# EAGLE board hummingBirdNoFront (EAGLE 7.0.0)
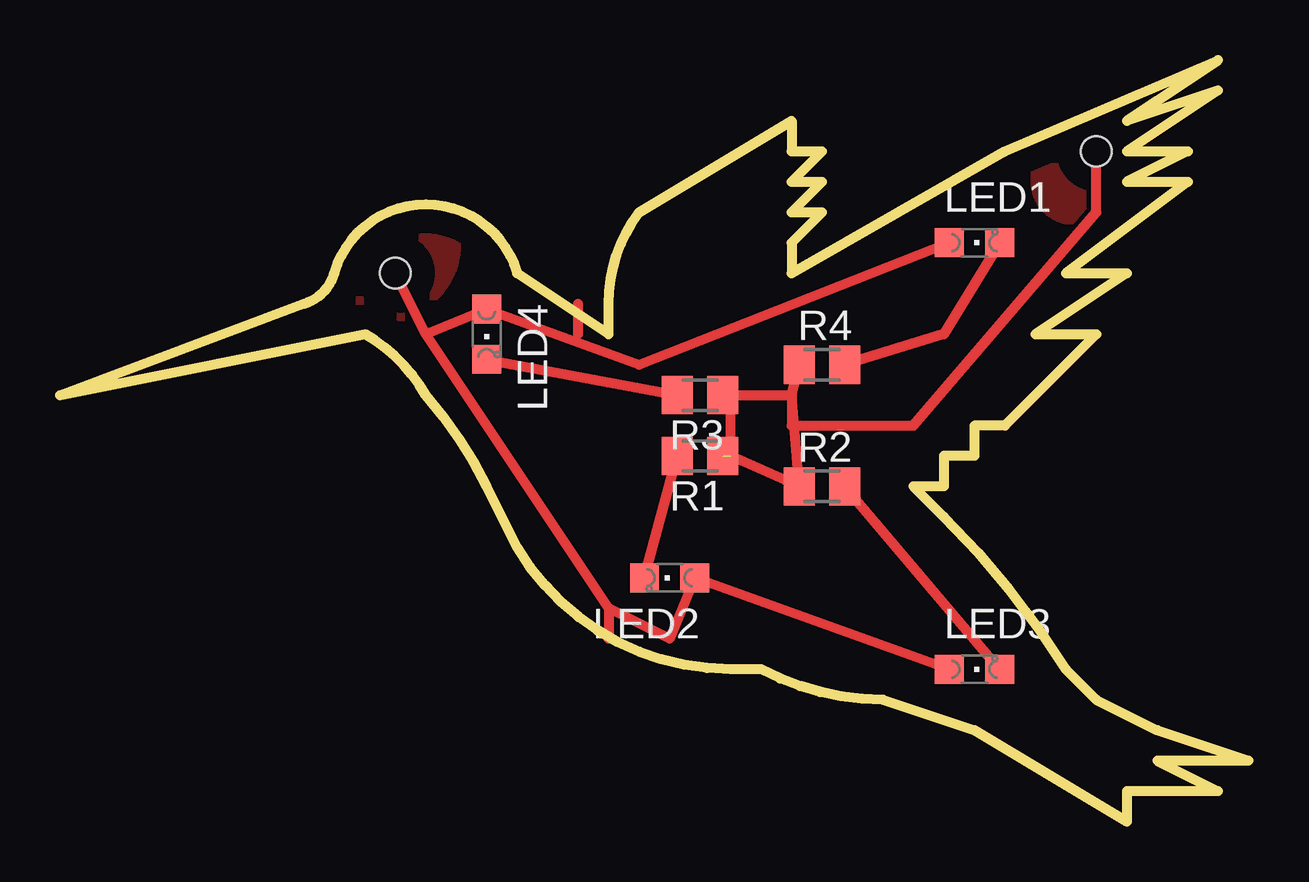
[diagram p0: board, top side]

Size 49.53 x 31.75 mm. Coordinates in mm from the lower left corner, seen from the top.
Outline: 0,17.78 10.16,21.59 arc58 11.43,22.86 arc-148 19.05,22.86 22.86,20.32 22.86,21.59 arc-37 24.13,25.4 30.48,29.21 30.48,27.94 31.75,27.94 30.48,26.67 31.75,26.67 30.48,25.4 31.75,25.4 30.48,24.13 30.48,22.86 39.37,27.94 48.26,31.75 44.45,29.21 48.26,30.48 44.45,27.94 46.99,27.94 44.45,26.67 46.99,26.67 41.91,22.86 44.45,22.86 40.64,20.32 43.18,20.32 39.37,16.51 38.1,16.51 38.1,15.24 36.83,15.24 36.83,13.97 35.56,13.97 36.83,12.7 arc-13 41.91,6.35 43.18,5.08 45.72,3.81 49.53,2.54 45.72,2.54 48.26,1.27 44.45,1.27 44.45,0 38.1,3.81 34.29,5.08 arc-28 29.21,6.35 27.94,6.35 arc-59 19.05,11.43 17.78,13.97 arc14 15.24,17.78 arc31 12.7,20.32 0,17.78
Copper layers (1*16): Top 0.035mm / dielectric 1.5mm / Bottom 0.035mm
Design rules "default": minimum track width 10mil, minimum drill 24mil, track to track 8mil, track to pad 8mil, pad to pad 8mil, via to via 8mil, smd to smd 8mil, copper to edge 40mil, drill to drill 8mil, minimum pad ring 10mil, minimum via ring 8mil, stop-mask expansion 4mil, vias tented up to drill 0mil, thermal gap 10mil
Holes 1.27 mm at 13.97,22.86 43.18,27.94

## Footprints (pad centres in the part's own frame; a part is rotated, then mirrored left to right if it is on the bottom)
CHIPLED_0805 = smd 1.2 x 1.2: A 0,-1.05; C 0,1.05
M0805 = smd 1.3 x 1.6: 1 -0.95,0; 2 0.95,0

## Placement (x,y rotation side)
LED1  [CHIPLED_0805]  38.1,24.13 270 top
LED2  [CHIPLED_0805]  25.4,10.16 90 top
LED3  [CHIPLED_0805]  38.1,6.35 270 top
LED4  [CHIPLED_0805]  17.78,20.32 180 top
R1  [M0805]  26.67,15.24 180 top
R2  [M0805]  31.75,13.97 0 top
R3  [M0805]  26.67,17.78 180 top
R4  [M0805]  31.75,19.05 0 top

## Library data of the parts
LED1-LED4 = led
R1-R4 = resistor

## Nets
N$1: LED1.A LED2.A LED3.A LED4.A
N$2: LED2.C R1.2
N$3: LED3.C R2.2
N$4: LED4.C R3.2
N$5: LED1.C R4.2
N$6: R1.1 R2.1 R3.1 R4.1

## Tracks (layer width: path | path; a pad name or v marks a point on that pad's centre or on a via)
N$1
  Top 0.406: LED1.A 24.13,19.05 LED4.A 15.24,20.32 | LED3.A LED2.A 25.4,7.62 22.86,8.89 | 22.86,8.89 15.24,20.32 | 15.24,20.32 13.97,22.86 | 22.86,8.89 22.86,7.62
N$2
  Top 0.406: LED2.C R1.2
N$3
  Top 0.406: LED3.C R2.2
N$4
  Top 0.406: LED4.C R3.2
N$5
  Top 0.406: LED1.C 36.83,20.32 R4.2
N$6  (1 unrouted)
  Top 0.406: R3.1 27.94,17.78 | 27.94,17.78 30.48,17.78 | 30.48,17.78 R4.1 | 30.48,17.78 R2.1 27.94,15.24 27.94,17.78 | 30.48,17.78 30.48,16.51 35.56,16.51 43.18,25.4 43.18,27.94
N$7
  Top 0.406: 21.59,20.32 21.59,21.59
N$8
  pour Top: 13.97,25.4 15.24,25.4 arc-90 16.51,24.13 arc-53 15.24,21.59 arc-21 12.7,20.32 arc-159 11.43,22.86 arc16
N$9
  pour Top: 40.64,27.94 40.64,26.67 arc127 43.18,25.4 arc-21 45.72,26.67 arc184 44.45,30.48 arc26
